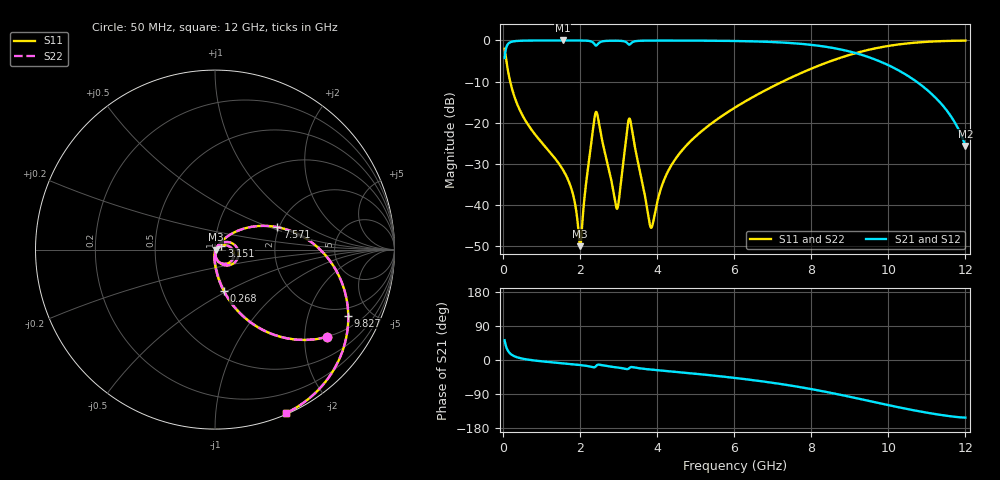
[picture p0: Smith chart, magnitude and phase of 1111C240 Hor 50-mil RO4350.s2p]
# GHz S MA R 50
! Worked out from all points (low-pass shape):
!   11951 points, 50 MHz to 12 GHz, reference 50 ohm
!   highest |S21| = -0.01 dB at 1.563 GHz (marker M1); lowest = -25.6 dB at 12 GHz (marker M2)
!   |S21| within 3 dB of the highest: 64.9 MHz to 9.127 GHz (9.062 GHz wide, 197 % of centre)
!   lowest |S11| = -50.0 dB at 2.011 GHz (marker M3), VSWR 1.01, Z = 50.3 - j0.119 ohm
!   |S11| at or under -10 dB: 194.2 MHz to 7.263 GHz (7.069 GHz wide, 190 % of centre)
!   |S22| runs from -50.0 to -0.1 dB; largest |S21 - S12| = 0
!   S11 on the Smith chart (normalised r, x): 50 MHz: 0.99, -2.58; 268 MHz: 0.99, -0.48; 3.151 GHz: 1.07, +0.04; 7.571 GHz: 1.96, +0.57; 9.827 GHz: 1.55, -3.65; 12 GHz: 0.01, -1.52
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0.05  0.7923 -37.9  0.61 52.1  0.61 52.1  0.7923 -37.9
0.15  0.3967 -67.6  0.9176 22.4  0.9176 22.4  0.3967 -67.6
0.268  0.2341 -78.1  0.9717 11.7  0.9717 11.7  0.2341 -78.1
1.563  0.02671 -96.3  0.9983 -8.9  0.9983 -8.9  0.02671 -96.3
1.815  0.01392 -94.1  0.9981 -11.3  0.9981 -11.3  0.01392 -94.1
2.011  0.00315 -22.1  0.9968 -13.3  0.9968 -13.3  0.00315 -22.1
2.042  0.004234 19.0  0.9963 -13.7  0.9963 -13.7  0.004234 19.0
2.187  0.02258 51.6  0.9909 -15.7  0.9909 -15.7  0.02258 51.6
2.412  0.1332 -9.6  0.8676 -17.0  0.8676 -17.0  0.1332 -9.6
2.948  0.009224 -38.4  0.9911 -19.3  0.9911 -19.3  0.009224 -38.4
3.151  0.04061 30.8  0.9751 -22.7  0.9751 -22.7  0.04061 30.8
3.301  0.1098 -38.4  0.8951 -19.7  0.8951 -19.7  0.1098 -38.4
3.824  0.005577 -38.3  0.9943 -25.0  0.9943 -25.0  0.005577 -38.3
4.034  0.01214 41.2  0.9952 -27.1  0.9952 -27.1  0.01214 41.2
4.656  0.04626 52.2  0.9948 -32.9  0.9948 -32.9  0.04626 52.2
6.025  0.1526 40.9  0.9833 -47.4  0.9833 -47.4  0.1526 40.9
7.571  0.3697 19.7  0.9215 -69.1  0.9215 -69.1  0.3697 19.7
8.017  0.456 11.9  0.8812 -77.0  0.8812 -77.0  0.456 11.9
9.827  0.8286 -26.4  0.5441 -115.3  0.5441 -115.3  0.8286 -26.4
10.009  0.8574 -30.4  0.498 -119.3  0.498 -119.3  0.8574 -30.4
11.258  0.9747 -55.0  0.1941 -143.3  0.1941 -143.3  0.9747 -55.0
12  0.9939 -66.6  0.05222 -152.0  0.05222 -152.0  0.9939 -66.6
